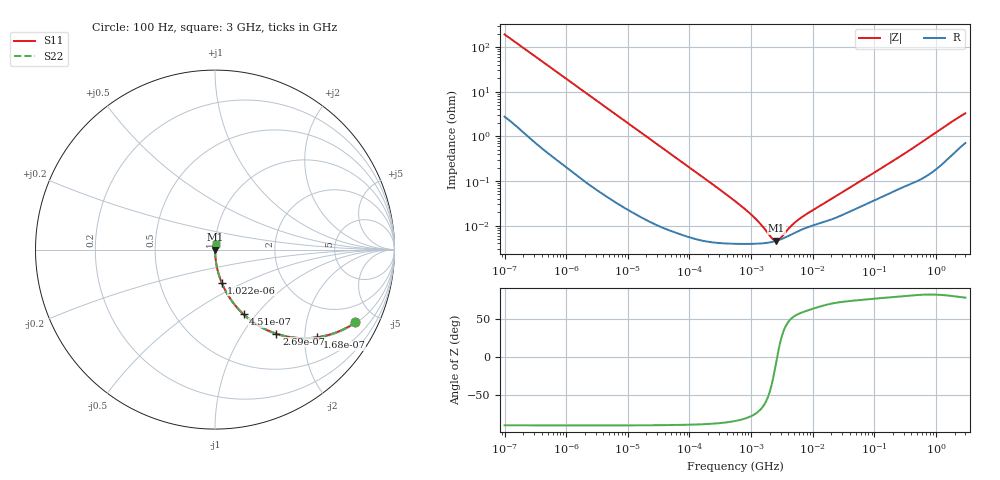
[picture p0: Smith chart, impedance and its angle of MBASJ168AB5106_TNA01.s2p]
! MBASJ168AB5106_TNA01  S-PARAMETER MODEL  ( Standard Model )
! Model Generated by TAIYO YUDEN Corporation (http://www.ty-top.com)
! Version 1.0
! TAIYO YUDEN Control No. 220601
! Copyright(c) 2012 TAIYO YUDEN CO.,LTD. All Rights Reserved.
! Product Description (link to TY-COMPAS)
! https://ds.yuden.co.jp/TYCOMPAS/or/detail?pn=MBASJ168AB5106KTNA01&u=M
! Products Name : Multilayer Ceramic Capacitors
! Characteristics :
!  Capacitance : 10 [uF] , Rated Voltage : 6.3 [V] , TCC : X5R
!  Case Size : 1.6 x 0.8 / 0.063 x 0.031 [mm/inch] , Thickness : 0.8 / 0.031 [mm/inch]
!  (Conditions: Temperature = 25 [degC] , DC Bias Voltage = 0 [V])
! External Node Assignments :
!  1  o---| |---o  2
! GND o---------o GND
! Frequency Range : 100Hz  -  3GHz  [ 401 STEP ]
# MHZ S RI R 50
! Freq[MHz].  S11 Real  S11 Imag  S21 Real  S21 Imag  S12 Real  S12 Imag  S22 Real  S22 Imag
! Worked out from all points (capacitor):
!   401 points, 100 Hz to 3 GHz, reference 50 ohm
!   read as one part in series: C = 8.28 uF near 109 Hz
!   lowest |Z| = 4.59 mohm at 2.579 MHz (marker M1)
!   series resonance near 2.648 MHz, so ESL is about 440 pH
!   S11 on the Smith chart (normalised r, x): 100 Hz: 1.06, -3.83; 168 Hz: 1.03, -2.30; 269 Hz: 1.02, -1.44; 451 Hz: 1.01, -0.86; 1.022 kHz: 1.00, -0.38; 3 GHz: 1.01, +0.06
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0.0001  0.7826 -0.4054  0.2174 0.4054  0.2174 0.4054  0.7826 -0.4054
0.000119  0.7204 -0.4418  0.2796 0.4418  0.2796 0.4418  0.7204 -0.4418
0.000168  0.5684 -0.4887  0.4316 0.4887  0.4316 0.4887  0.5684 -0.4887
0.000208  0.4636 -0.4924  0.5364 0.4924  0.5364 0.4924  0.4636 -0.4924
0.000269  0.3425 -0.4686  0.6575 0.4686  0.6575 0.4686  0.3425 -0.4686
0.000451  0.159 -0.3602  0.841 0.3602  0.841 0.3602  0.159 -0.3602
0.000664  0.0814 -0.2682  0.9186 0.2682  0.9186 0.2682  0.0814 -0.2682
0.001022  0.0369 -0.1835  0.9631 0.1835  0.9631 0.1835  0.0369 -0.1835
0.001788  0.0129 -0.108  0.9871 0.108  0.9871 0.108  0.0129 -0.108
0.005476  0.00167 -0.0359  0.9983 0.0359  0.9983 0.0359  0.00167 -0.0359
0.031977  0.000136 -0.00623  0.9999 0.00623  0.9999 0.00623  0.000136 -0.00623
0.547723  3.93e-05 -0.000353  1 0.000353  1 0.000353  3.93e-05 -0.000353
0.918067  3.9e-05 -0.000194  1 0.000194  1 0.000194  3.9e-05 -0.000194
1.473992  4e-05 -9.46e-05  1 9.46e-05  1 9.46e-05  4e-05 -9.46e-05
1.677156  4.06e-05 -7.21e-05  1 7.21e-05  1 7.21e-05  4.06e-05 -7.21e-05
2.579298  4.57e-05 -3.92e-06  1 3.92e-06  1 3.92e-06  4.57e-05 -3.92e-06
4.513443  6.37e-05 7.7e-05  0.9999 -7.7e-05  0.9999 -7.7e-05  6.37e-05 7.7e-05
6.648799  8.18e-05 0.000132  0.9999 -0.000132  0.9999 -0.000132  8.18e-05 0.000132
9.794414  9.97e-05 0.000194  0.9999 -0.000194  0.9999 -0.000194  9.97e-05 0.000194
175.1444  0.000535 0.00245  0.9995 -0.00245  0.9995 -0.00245  0.000535 0.00245
1789.813  0.00414 0.0206  0.9959 -0.0206  0.9959 -0.0206  0.00414 0.0206
3000  0.00806 0.0317  0.9919 -0.0317  0.9919 -0.0317  0.00806 0.0317
